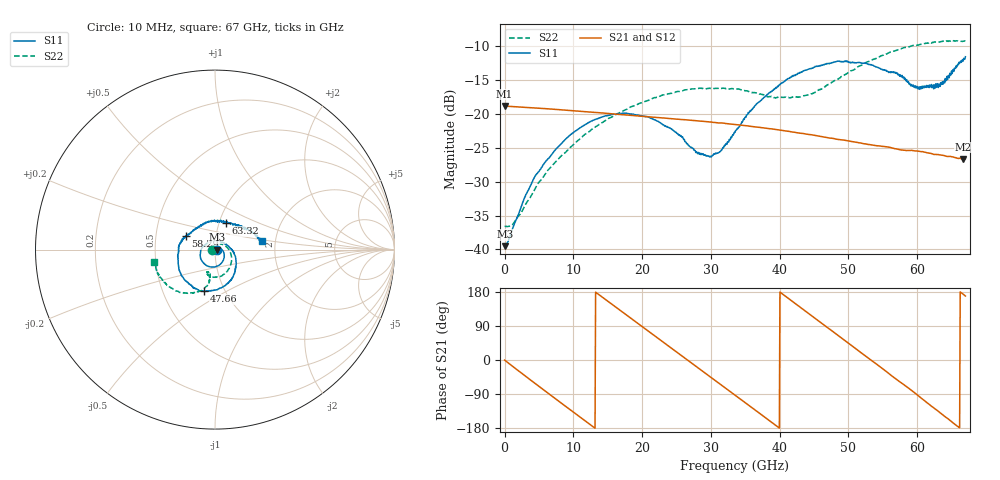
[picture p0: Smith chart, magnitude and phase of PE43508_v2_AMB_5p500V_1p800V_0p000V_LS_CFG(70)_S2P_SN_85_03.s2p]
!Keysight Technologies,N5227A,US51270237,A.10.43.00
!Date: Wednesday, August 22, 2018 17:13:55
!Correction: S11(Full 2 Port(1,3))
!S31(Full 2 Port(1,3))
!S13(Full 2 Port(1,3))
!S33(Full 2 Port(1,3))
!S2P File: Measurements: S11, S31, S13, S33:
# Hz S  dB  R 50
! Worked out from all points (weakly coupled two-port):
!   801 points, 10 MHz to 67 GHz, reference 50 ohm
!   highest |S21| = -18.85 dB at 10 MHz (marker M1); lowest = -26.7 dB at 66.67 GHz (marker M2)
!   lowest |S11| = -39.5 dB at 93.74 MHz (marker M3), VSWR 1.02, Z = 51.1 + j0.0385 ohm
!   |S11| at or under -10 dB: start of sweep to end of sweep
!   |S22| runs from -36.6 to -9.2 dB; largest |S21 - S12| = 0.00059
!   S11 on the Smith chart (normalised r, x): 10 MHz: 1.02, -0.00; 47.66 GHz: 0.80, -0.39; 58.29 GHz: 0.71, +0.11; 63.32 GHz: 1.07, +0.33; 67 GHz: 1.69, +0.17
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1e7  -39.40 -1.7  -18.85 -0.2  -18.85 -0.2  -36.64 -179.7
9.37375e7  -39.52 2.0  -18.86 -1.4  -18.87 -1.5  -36.59 176.8
1.3498e9  -36.42 19.4  -18.95 -19.2  -18.95 -19.2  -36.09 137.6
4.531825e9  -29.07 5.3  -19.14 -63.1  -19.15 -63.1  -30.89 75.5
7.546375e9  -25.14 -23.9  -19.36 -104.3  -19.36 -104.2  -26.95 43.6
1.123082e10  -21.88 -60.0  -19.64 -154.1  -19.64 -154.1  -23.46 11.2
1.725992e10  -19.90 -114.3  -20.14 125.0  -20.14 125.1  -19.54 -28.7
2.236791e10  -21.15 -159.8  -20.56 56.8  -20.55 56.7  -17.50 -56.1
2.797832e10  -25.67 125.5  -21.03 -18.3  -21.04 -18.3  -16.30 -81.2
2.973681e10  -26.29 90.1  -21.19 -41.9  -21.19 -41.9  -16.22 -88.2
3.132782e10  -25.57 56.2  -21.35 -63.1  -21.36 -63.1  -16.24 -94.2
3.3505e10  -22.75 18.4  -21.58 -92.7  -21.59 -92.7  -16.34 -101.2
3.836178e10  -17.04 -33.1  -22.18 -158.1  -22.19 -158.0  -17.47 -108.8
4.472582e10  -13.28 -83.0  -23.10 115.8  -23.10 115.8  -17.03 -101.2
4.765664e10  -12.46 -105.1  -23.61 76.1  -23.60 76.0  -15.33 -100.4
5.15923e10  -12.45 -135.0  -24.27 22.6  -24.25 22.6  -12.95 -105.3
5.586291e10  -13.91 -176.5  -24.91 -35.7  -24.89 -36.1  -10.99 -120.4
5.82913e10  -14.91 155.0  -25.40 -68.4  -25.40 -68.7  -10.20 -129.8
6.004979e10  -15.97 125.9  -25.48 -92.8  -25.49 -93.2  -9.89 -137.3
6.331555e10  -15.96 68.3  -26.05 -139.1  -26.09 -139.6  -9.39 -151.9
6.666505e10  -12.24 15.5  -26.66 173.9  -26.73 173.9  -9.28 -166.4
6.7e10  -11.58 10.4  -26.66 168.8  -26.74 168.8  -9.26 -168.2
